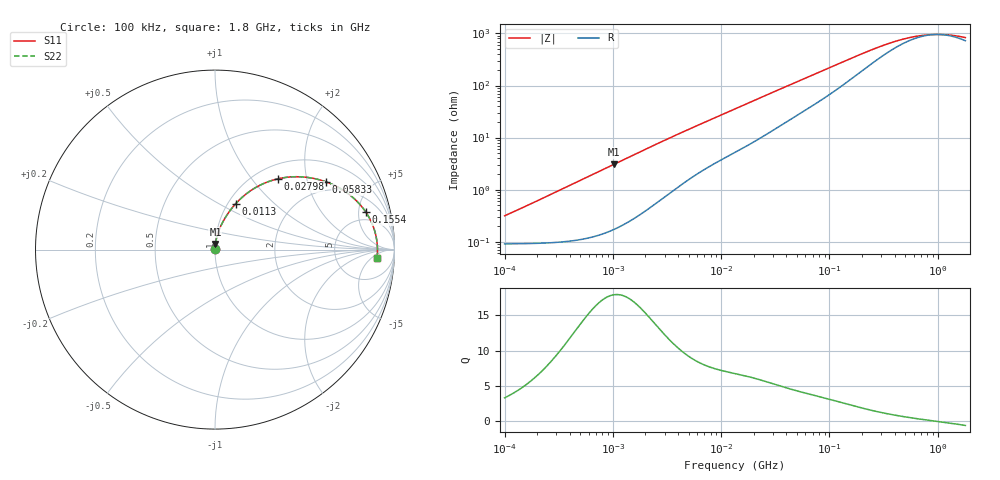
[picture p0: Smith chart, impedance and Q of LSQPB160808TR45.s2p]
! LSQPB160808TR45  S-PARAMETER MODEL  ( General Type )
! Model Generated by TAIYO YUDEN Corporation (http://www.ty-top.com)
! Version 4.0
! TAIYO YUDEN Control No. 100810NF18SB-HKC
! Copyright(c) 2007 TAIYO YUDEN CO.,LTD. All Rights Reserved.
! Product Description (link to TY-COMPAS)
! https://ds.yuden.co.jp/TYCOMPAS/or/detail?pn=LSQPB160808TR45M&u=M
! Products Name : Inductors
! Characteristics :
!  Inductance : 0.45 uH , SRF(min) : 200 MHz , DC Resistance(max) : 0.117 Ohm
!  Rated Current : Saturation :1250 mA , Temp Rise : 800 mA (40 degC)
!  Case Size : 1.6 x 0.8 / 0.063 x 0.031 [mm/inch] , Thickness : 0.8 / 0.031 [mm/inch]
!  (Conditions: Temperature = 25 degC , DC Bias Current/Voltage = 0A / 0V)
! External Node Assignments :
!  1  o---GGG---o  2
! GND o---------o GND
! Frequency Range : 0.1MHz  -  1800MHz  [ 402 STEP ]
# MHz S RI R 50
! Freq[MHz].  S11 Real  S11 Imag  S21 Real  S21 Imag  S12 Real  S12 Imag  S22 Real  S22 Imag
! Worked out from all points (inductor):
!   401 points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, 100 kHz to 1.8 GHz, reference 50 ohm
!   read as one part in series: L = 480 nH near 105 kHz
!   highest Q = 17.9 at 1.025 MHz (marker M1), where L = 478 nH
!   self-resonance near 984.7 MHz
!   S11 on the Smith chart (normalised r, x): 100 kHz: 1.00, +0.01; 11.3 MHz: 1.09, +0.60; 27.98 MHz: 1.25, +1.37; 58.33 MHz: 1.65, +2.62; 155.4 MHz: 3.58, +6.00; 1.8 GHz: 15, -8
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0.1  0.000916 0.00301  0.9991 -0.00301  0.9991 -0.00301  0.000916 0.00301
0.159267  0.000942 0.00479  0.9991 -0.00479  0.9991 -0.00479  0.000942 0.00479
0.516129  0.00135 0.0155  0.9986 -0.0155  0.9986 -0.0155  0.00135 0.0155
1.024772  0.00266 0.0307  0.9973 -0.0307  0.9973 -0.0307  0.00266 0.0307
2.66389  0.012 0.0774  0.988 -0.0774  0.988 -0.0774  0.012 0.0774
5.97828  0.0455 0.1576  0.9545 -0.1576  0.9545 -0.1576  0.0455 0.1576
8.423854  0.0757 0.2061  0.9243 -0.2061  0.9243 -0.2061  0.0757 0.2061
11.30236  0.1144 0.2547  0.8856 -0.2547  0.8856 -0.2547  0.1144 0.2547
13.41641  0.1444 0.2851  0.8556 -0.2851  0.8556 -0.2851  0.1444 0.2851
19.37354  0.2321 0.3489  0.7679 -0.3489  0.7679 -0.3489  0.2321 0.3489
27.97575  0.3516 0.3946  0.6484 -0.3946  0.6484 -0.3946  0.3516 0.3946
40.39749  0.488 0.4049  0.512 -0.4049  0.512 -0.4049  0.488 0.4049
58.33472  0.6185 0.3775  0.3815 -0.3775  0.3815 -0.3775  0.6185 0.3775
69.24595  0.6723 0.3545  0.3277 -0.3545  0.3277 -0.3545  0.6723 0.3545
102.472  0.7716 0.2875  0.2284 -0.2875  0.2284 -0.2875  0.7716 0.2875
155.4012  0.8393 0.2105  0.1607 -0.2105  0.1607 -0.2105  0.8393 0.2105
224.4022  0.873 0.1499  0.127 -0.1499  0.127 -0.1499  0.873 0.1499
357.3983  0.8939 0.0892  0.1061 -0.0892  0.1061 -0.0892  0.8939 0.0892
555.4434  0.9022 0.0457  0.0978 -0.0457  0.0978 -0.0457  0.9022 0.0457
821.96  0.9049 0.0138  0.0951 -0.0138  0.0951 -0.0138  0.9049 0.0138
1186.925  0.9052 -0.0143  0.0948 0.0143  0.0948 0.0143  0.9052 -0.0143
1800  0.9029 -0.0486  0.0971 0.0486  0.0971 0.0486  0.9029 -0.0486
